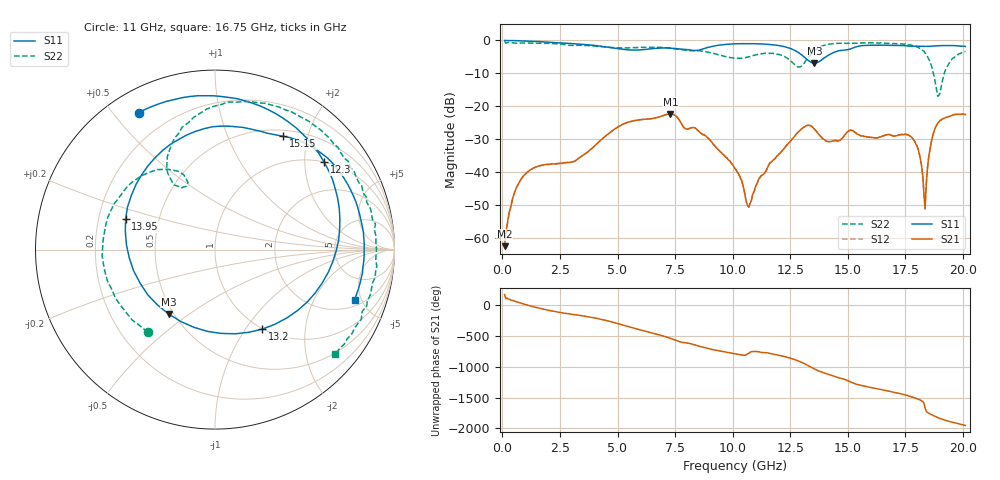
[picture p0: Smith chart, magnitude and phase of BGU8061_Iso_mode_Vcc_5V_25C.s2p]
# GHZ S DB R 50
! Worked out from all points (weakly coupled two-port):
!   401 points, 100 MHz to 20.1 GHz, reference 50 ohm
!   highest |S21| = -22.41 dB at 7.3 GHz (marker M1); lowest = -62.4 dB at 100 MHz (marker M2)
!   lowest |S11| = -7.1 dB at 13.55 GHz (marker M3), VSWR 2.58, Z = 23.5 - j21 ohm
!   |S11| at or under -10 dB: nowhere
!   |S22| runs from -17.1 to -0.5 dB; largest |S21 - S12| = 0.0016
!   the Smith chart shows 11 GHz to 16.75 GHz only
!   S11 on the Smith chart (normalised r, x): 11 GHz: 0.09, +0.58; 12.3 GHz: 1.01, +2.50; 13.2 GHz: 0.99, -1.20; 13.95 GHz: 0.32, +0.15; 15.15 GHz: 0.58, +1.61; 16.75 GHz: 2.45, -4.37
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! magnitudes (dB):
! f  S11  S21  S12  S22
! 100 MHz  -0.2  -62.4  -59.0  -0.5
! 500 MHz  -0.2  -46.8  -46.9  -0.9
! 950 MHz  -0.4  -41.0  -41.0  -1.0
! 3.45 GHz  -1.4  -35.2  -35.2  -1.6
! 5.2 GHz  -2.8  -25.7  -25.7  -2.4
! 6.8 GHz  -2.5  -23.3  -23.3  -2.2
! 7.3 GHz  -2.5  -22.4  -22.4  -2.5
! 10.1 GHz  -1.2  -38.9  -39.0  -5.5
! 10.65 GHz  -1.2  -50.2  -50.1  -5.2
! 11 GHz  -1.2  -44.2  -44.3  -4.5
! 12.3 GHz  -2.2  -32.2  -32.3  -5.2
! 13.2 GHz  -5.8  -25.9  -26.0  -6.0
! 13.45 GHz  -7.0  -26.3  -26.3  -3.9
! 13.55 GHz  -7.1  -27.0  -27.0  -3.3
! 13.95 GHz  -5.6  -30.1  -30.1  -1.7
! 15.15 GHz  -2.7  -27.4  -27.4  -1.1
! 16.75 GHz  -1.7  -28.6  -28.6  -1.0
! 16.8 GHz  -1.7  -28.6  -28.6  -1.1
! 17.85 GHz  -1.9  -30.3  -30.2  -1.7
! 18.35 GHz  -2.0  -51.1  -51.2  -4.0
! 18.85 GHz  -1.8  -25.8  -25.9  -15.2
! 20.1 GHz  -2.0  -22.6  -22.6  -3.5
